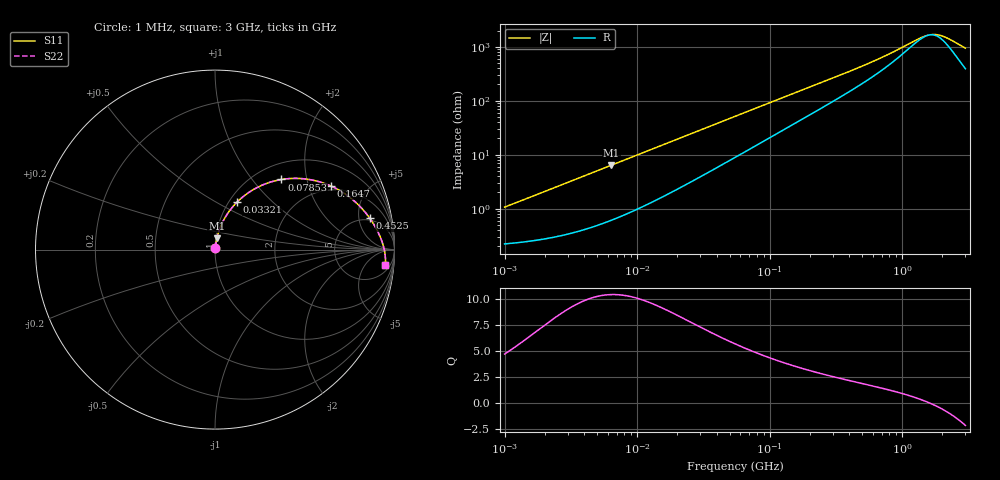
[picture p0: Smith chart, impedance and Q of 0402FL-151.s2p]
# MHz S MA R 50
!Freq  MagS11  AngS11  MagS21  AngS21  MagS12  AngS12  MagS22  AngS22
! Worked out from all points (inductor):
!   801 points, 1 MHz to 3 GHz, reference 50 ohm
!   read as one part in series: L = 165 nH near 1.041 MHz
!   highest Q = 10.4 at 6.369 MHz (marker M1), where L = 159 nH
!   self-resonance near 1.597 GHz
!   S11 on the Smith chart (normalised r, x): 1 MHz: 1.00, +0.02; 33.21 MHz: 1.09, +0.63; 78.53 MHz: 1.29, +1.42; 164.7 MHz: 1.83, +2.83; 452.5 MHz: 4.57, +7.07; 3 GHz: 9, -17
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1  0.01067 77.4  0.9977 -0.6  0.9977 -0.6  0.01067 77.4
3.823119  0.03869 81.9  0.9953 -2.2  0.9953 -2.2  0.03869 81.9
6.369191  0.06332 80.9  0.992 -3.6  0.992 -3.6  0.06332 80.9
14.47069  0.1382 76.0  0.9758 -7.9  0.9758 -7.9  0.1382 76.0
22.70269  0.2089 71.0  0.9527 -12.0  0.9527 -12.0  0.2089 71.0
33.20783  0.2905 65.2  0.9168 -16.7  0.9168 -16.7  0.2905 65.2
42.64819  0.3554 60.5  0.8809 -20.6  0.8809 -20.6  0.3554 60.5
54.77226  0.4277 55.1  0.8329 -24.9  0.8329 -24.9  0.4277 55.1
78.52918  0.5381 46.5  0.7411 -31.8  0.7411 -31.8  0.5381 46.5
112.5904  0.6439 37.6  0.6278 -38.7  0.6278 -38.7  0.6439 37.6
164.6891  0.7375 28.7  0.4996 -45.1  0.4996 -45.1  0.7375 28.7
209.4008  0.7843 23.6  0.4221 -48.2  0.4221 -48.2  0.7843 23.6
303.2461  0.8392 17.1  0.3157 -51.2  0.3157 -51.2  0.8392 17.1
452.5341  0.8799 11.4  0.2223 -51.8  0.2223 -51.8  0.8799 11.4
611.0031  0.9018 8.1  0.1662 -49.8  0.1662 -49.8  0.9018 8.1
792.5923  0.9165 5.6  0.1256 -45.6  0.1256 -45.6  0.9165 5.6
1374.365  0.9386 1.2  0.0644 -17.0  0.0644 -17.0  0.9386 1.2
1534.307  0.9419 0.3  0.05836 -5.0  0.05836 -5.0  0.9419 0.3
1678.92  0.9443 -0.4  0.0561 6.5  0.0561 6.5  0.9443 -0.4
1855.641  0.9467 -1.2  0.05687 19.8  0.05687 19.8  0.9467 -1.2
2071.593  0.949 -2.0  0.06174 33.3  0.06174 33.3  0.949 -2.0
3000  0.9537 -5.3  0.1012 60.2  0.1012 60.2  0.9537 -5.3
